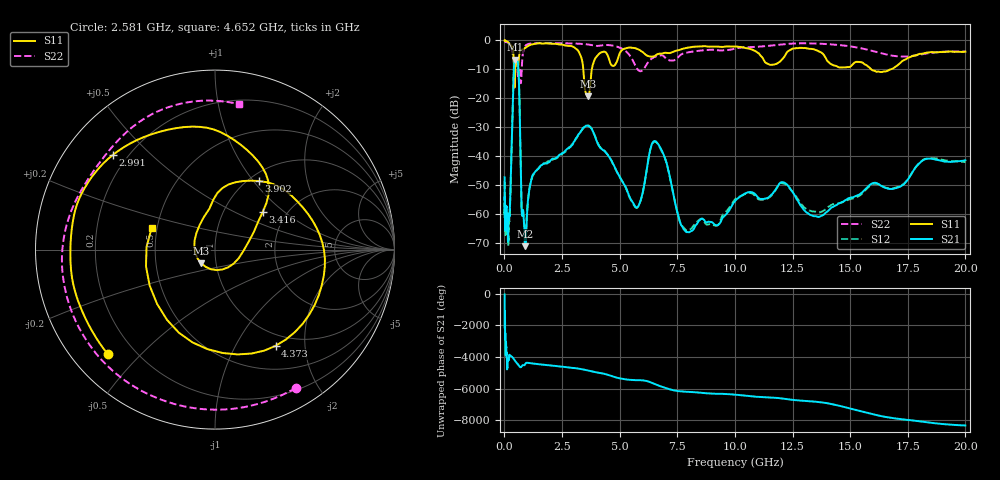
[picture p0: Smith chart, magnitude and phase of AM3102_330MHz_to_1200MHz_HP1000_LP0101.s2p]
! Date/Time: Tue, Sep 11, 2018 5:17 PM
! Network Analyzer: Agilent Technologies E8362B Rev: A.07.50.63
! Sweep from 0.010 to 20.000 GHz, 1601 Points, Sweep Type: LOG
! Power Supply: 4.949 V, 0.001 A
# Hz S DB R 50
!freq MagS11 AngS11 MagS21 AngS21 MagS12 AngS12 MagS22 AngS22
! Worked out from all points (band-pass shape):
!   1601 points, 10 MHz to 20 GHz, reference 50 ohm
!   highest |S21| = -6.68 dB at 458 MHz (marker M1); lowest = -71.2 dB at 912 MHz (marker M2)
!   |S21| within 3 dB of the highest: 412.4 MHz to 606.5 MHz (194.1 MHz wide, 38.1 % of centre)
!   lowest |S11| = -19.3 dB at 3.617 GHz (marker M3), VSWR 1.24, Z = 42.4 - j6.55 ohm
!   |S11| at or under -10 dB: 415.9 MHz to 467.6 MHz (51.62 MHz wide, 11.7 % of centre); 3.423 GHz to 3.792 GHz (369.2 MHz wide, 10.2 % of centre); 15.91 GHz to 16.76 GHz (850.1 MHz wide, 5.2 % of centre)
!   |S22| runs from -14.8 to -0.1 dB; largest |S21 - S12| = 0.0071
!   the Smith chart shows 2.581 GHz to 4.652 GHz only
!   S11 on the Smith chart (normalised r, x): 2.581 GHz: 0.11, -0.40; 2.991 GHz: 0.15, +0.39; 3.416 GHz: 1.52, +0.72; 3.902 GHz: 1.11, +1.06; 4.373 GHz: 0.82, -1.48; 4.652 GHz: 0.47, +0.13
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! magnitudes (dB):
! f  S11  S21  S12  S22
! 10 MHz  0.0  -47.4  -48.9  -0.1
! 35.55 MHz  0.0  -62.6  -62.2  -0.3
! 126.4 MHz  -0.4  -63.2  -64.8  -0.8
! 238.9 MHz  -1.1  -57.9  -58.8  -1.4
! 447.2 MHz  -15.8  -6.8  -6.8  -7.2
! 458 MHz  -12.9  -6.7  -6.7  -6.9
! 609 MHz  -8.0  -10.0  -10.1  -12.7
! 750.6 MHz  -3.1  -58.8  -58.6  -10.3
! 912 MHz  -2.5  -71.2  -70.8  -1.8
! 1.103 GHz  -1.6  -50.6  -50.4  -1.1
! 1.59 GHz  -1.0  -43.2  -43.3  -0.9
! 2.581 GHz  -1.6  -38.8  -38.8  -1.0
! 2.991 GHz  -2.2  -35.4  -35.4  -1.0
! 3.416 GHz  -9.4  -30.2  -30.5  -1.2
! 3.617 GHz  -19.3  -29.5  -29.3  -1.4
! 3.902 GHz  -6.9  -32.6  -32.5  -1.8
! 4.373 GHz  -4.0  -38.5  -38.5  -1.6
! 4.652 GHz  -8.6  -41.7  -41.8  -1.7
! 5.652 GHz  -2.6  -57.2  -57.4  -8.2
! 6.549 GHz  -5.2  -34.8  -35.0  -5.6
! 7.958 GHz  -2.5  -66.3  -65.7  -4.1
! 20 GHz  -3.9  -41.5  -42.1  -3.8
